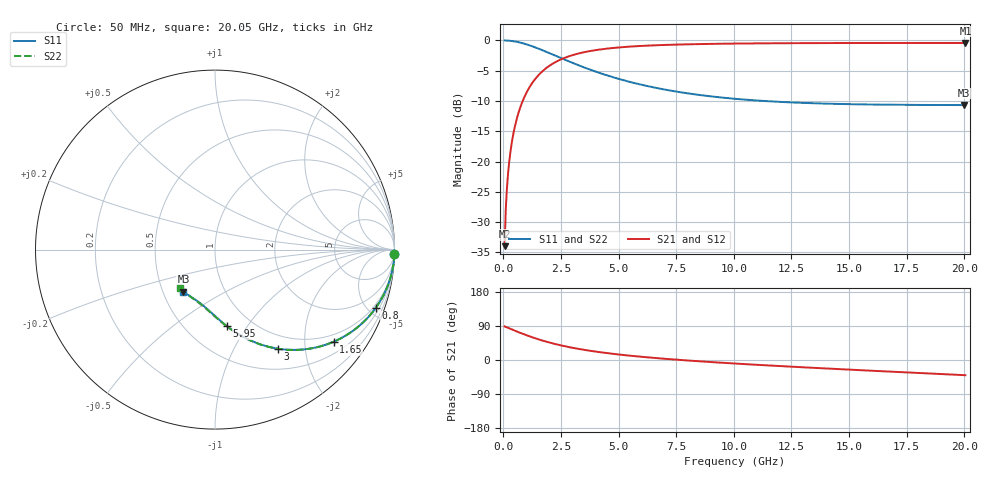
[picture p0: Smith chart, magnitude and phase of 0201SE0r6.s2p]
! AVX Thin Film Operation		Date: August 2001
! Description: Accu-P® Series, Thin Film, SMD, RF Capacitor
! Part Number: 02013J0R6ABW
! 50 MHz  -  20.05 GHz
! Serial Measurements
# mhz S db R 50
!	S11		S21		S12		S22
!	dB	Phase	dB	Phase	dB	Phase	dB	Phase
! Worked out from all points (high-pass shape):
!   401 points, 50 MHz to 20.05 GHz, reference 50 ohm
!   highest |S21| = -0.41 dB at 20.05 GHz (marker M1); lowest = -34.0 dB at 50 MHz (marker M2)
!   |S21| within 3 dB of the highest: 2.336 GHz to end of sweep
!   lowest |S11| = -10.7 dB at 20 GHz (marker M3), VSWR 1.83, Z = 31.8 - j16.3 ohm
!   |S11| at or under -10 dB: 11.34 GHz to end of sweep
!   |S22| runs from -10.7 to 0.0 dB; largest |S21 - S12| = 0
!   S11 on the Smith chart (normalised r, x): 50 MHz: 1, -89; 800 MHz: 0.79, -5.56; 1.65 GHz: 0.79, -2.71; 3 GHz: 0.79, -1.51; 5.95 GHz: 0.77, -0.81; 20.05 GHz: 0.64, -0.32
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50  -0.00 -1.3  -33.96 88.7  -33.96 88.7  -0.00 -1.3
100  -0.01 -2.6  -27.95 87.4  -27.95 87.4  -0.01 -2.6
200  -0.03 -5.2  -21.95 84.8  -21.95 84.8  -0.03 -5.2
250  -0.04 -6.4  -20.03 83.6  -20.03 83.6  -0.04 -6.4
350  -0.09 -9.0  -17.15 81.0  -17.15 81.0  -0.09 -9.0
450  -0.14 -11.5  -15.02 78.5  -15.02 78.5  -0.14 -11.5
550  -0.21 -14.0  -13.35 76.0  -13.35 76.0  -0.21 -14.0
800  -0.42 -20.0  -10.32 70.0  -10.32 70.0  -0.42 -20.0
1200  -0.90 -29.0  -7.30 61.0  -7.30 61.0  -0.90 -29.0
1650  -1.55 -37.9  -5.24 52.1  -5.24 52.1  -1.55 -37.9
2250  -2.51 -47.8  -3.59 42.1  -3.59 42.1  -2.51 -47.9
3000  -3.71 -57.7  -2.42 32.2  -2.42 32.2  -3.71 -57.7
3400  -4.31 -62.0  -2.02 27.8  -2.02 27.8  -4.31 -62.1
4550  -5.83 -72.0  -1.33 17.8  -1.33 17.8  -5.83 -72.2
5950  -7.28 -81.0  -0.91 8.7  -0.91 8.7  -7.28 -81.3
6750  -7.93 -85.1  -0.78 4.5  -0.78 4.5  -7.93 -85.6
8250  -8.87 -91.8  -0.62 -2.4  -0.62 -2.4  -8.88 -92.5
10050  -9.63 -98.4  -0.52 -9.4  -0.52 -9.4  -9.65 -99.7
13400  -10.37 -109.0  -0.44 -20.5  -0.44 -20.5  -10.39 -111.3
16750  -10.61 -118.3  -0.42 -30.6  -0.42 -30.6  -10.65 -122.0
20000  -10.67 -126.9  -0.41 -40.0  -0.41 -40.0  -10.71 -132.0
20050  -10.67 -127.1  -0.41 -40.1  -0.41 -40.1  -10.72 -132.1
